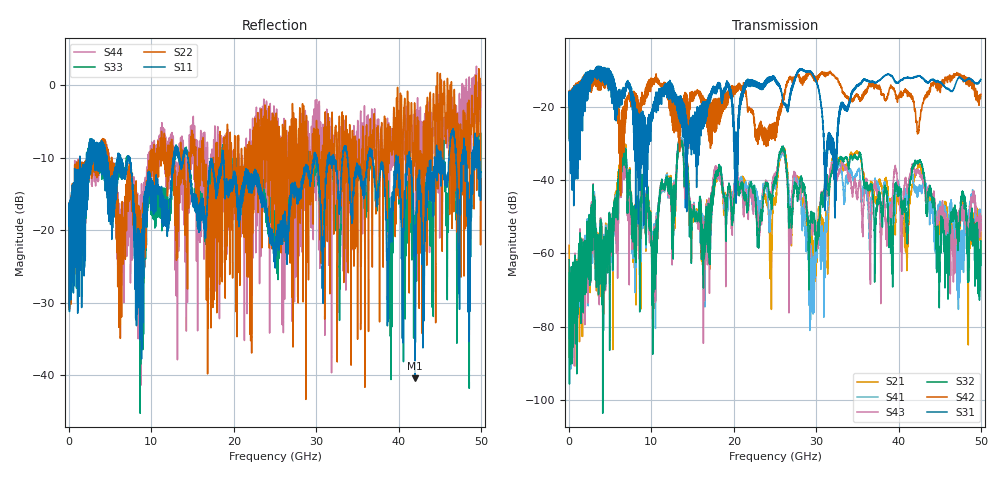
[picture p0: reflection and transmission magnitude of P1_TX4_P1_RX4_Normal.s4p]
!Keysight Technologies,N5225B,MY57041031,A.13.20.10
!Date: Friday, May 31, 2019 11:19:07
!Correction: S11(Full 4 Port(1,2,3,4))
!S12(Full 4 Port(1,2,3,4))
!S13(Full 4 Port(1,2,3,4))
!S14(Full 4 Port(1,2,3,4))
!S21(Full 4 Port(1,2,3,4))
!S22(Full 4 Port(1,2,3,4))
!S23(Full 4 Port(1,2,3,4))
!S24(Full 4 Port(1,2,3,4))
!S31(Full 4 Port(1,2,3,4))
!S32(Full 4 Port(1,2,3,4))
!S33(Full 4 Port(1,2,3,4))
!S34(Full 4 Port(1,2,3,4))
!S41(Full 4 Port(1,2,3,4))
!S42(Full 4 Port(1,2,3,4))
!S43(Full 4 Port(1,2,3,4))
!S44(Full 4 Port(1,2,3,4))
!S4P File: Measurements: <S11,S12,S13,S14>,
!<S21,S22,S23,S24>,
!<S31,S32,S33,S34>,
!<S41,S42,S43,S44>:
# Hz S  dB  R 50.0
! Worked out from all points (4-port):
!   5000 points, 10 MHz to 50 GHz, reference 50 ohm
!   strongest paths, dB at 10 MHz, 12.51 GHz, 25.01 GHz, 37.51 GHz, 50 GHz:
!     S31: -19.6, -17.6, -13.0, -13.0, -12.6
!     S42: -19.4, -19.4, -26.0, -14.9, -16.7
!     S32: -61.8, -48.6, -40.5, -46.3, -63.3
!     S43: -68.0, -51.4, -39.2, -43.6, -52.0
!     S41: -65.4, -49.9, -42.2, -41.0, -50.9
!     S21: -57.8, -47.9, -46.4, -42.4, -59.8
!   lowest |S11| = -40.4 dB at 42 GHz (marker M1), VSWR 1.02, Z = 49.2 + j0.509 ohm
!   |S11| at or under -10 dB: 7.336 GHz to 12.7 GHz (5.362 GHz wide, 53.5 % of centre); 14.41 GHz to 18.57 GHz (4.158 GHz wide, 25.2 % of centre); 18.74 GHz to 29.76 GHz (11.02 GHz wide, 45.4 % of centre)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
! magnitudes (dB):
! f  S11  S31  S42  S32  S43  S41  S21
! 10 MHz  -19.4  -19.6  -19.4  -61.8  -68.0  -65.4  -57.8
! 6.69 GHz  -12.9  -14.8  -25.0  -32.6  -36.0  -33.9  -31.5
! 10.29 GHz  -14.4  -19.4  -13.6  -54.2  -53.5  -52.8  -54.7
! 25.96 GHz  -19.3  -18.2  -19.0  -31.3  -31.8  -32.3  -31.4
! 29.42 GHz  -12.6  -10.6  -11.1  -48.6  -50.4  -71.3  -56.7
! 42 GHz  -40.4  -11.9  -20.8  -35.5  -37.5  -43.0  -39.0
! 50 GHz  -12.0  -12.6  -16.7  -63.3  -52.0  -50.9  -59.8
